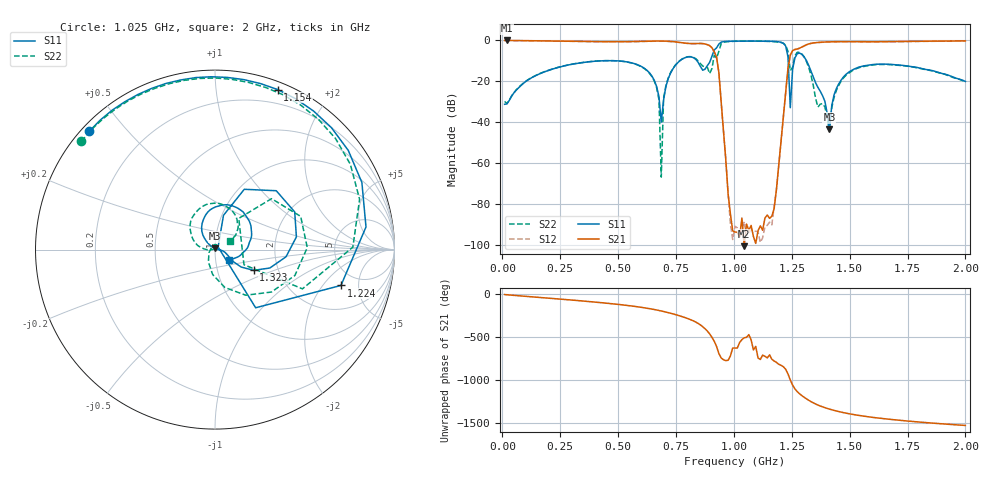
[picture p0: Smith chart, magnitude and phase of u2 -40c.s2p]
!Agilent Technologies,E8363B,SG43030131,A.07.50.48
!Agilent E8363B: A.07.50.48
!Date: Tuesday, December 02, 2025 02:29:57
!Correction: S11(Full 2 Port(1,2))
!S21(Full 2 Port(1,2))
!S12(Full 2 Port(1,2))
!S22(Full 2 Port(1,2))
!S2P File: Measurements: S11, S21, S12, S22:
# Hz S  dB  R 50
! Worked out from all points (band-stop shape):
!   201 points, 10 MHz to 2 GHz, reference 50 ohm
!   highest |S21| = 0.00 dB at 19.95 MHz (marker M1); lowest = -100.8 dB at 1.045 GHz (marker M2)
!   |S21| within 3 dB of the highest: start of sweep to 900.1 MHz; 1.297 GHz to end of sweep
!   lowest |S11| = -43.5 dB at 1.413 GHz (marker M3), VSWR 1.01, Z = 49.9 + j0.662 ohm
!   |S11| at or under -10 dB: start of sweep to 421.7 MHz; 498.7 MHz to 766.5 MHz (267.8 MHz wide, 42.3 % of centre); 1.314 GHz to end of sweep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
!   |S22| runs from -66.9 to -0.4 dB; largest |S21 - S12| = 0.019
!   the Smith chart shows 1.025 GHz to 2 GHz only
!   S11 on the Smith chart (normalised r, x): 1.025 GHz: 0.02, +0.40; 1.154 GHz: 0.07, +1.46; 1.224 GHz: 3.63, -3.10; 1.323 GHz: 1.49, -0.37; 2 GHz: 1.16, -0.14
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1e7  -31.26 -83.7  -0.01 -0.6  -0.08 -1.6  -29.86 -81.1
1.995e7  -31.10 -84.9  0.00 -3.4  -0.08 -4.1  -30.90 -87.6
3.483e8  -10.81 -166.1  -0.47 -76.1  -0.55 -76.1  -10.76 -163.3
6.7665e8  -27.61 91.5  -0.28 173.3  -0.35 173.3  -28.97 86.9
6.866e8  -39.99 135.0  -0.28 167.5  -0.35 167.5  -66.92 -45.5
6.9655e8  -29.17 -128.6  -0.30 161.4  -0.37 161.4  -28.30 -104.4
7.264e8  -16.06 -137.6  -0.46 141.4  -0.53 141.3  -15.84 -123.8
8.5575e8  -12.76 57.1  -1.45 3.8  -1.53 3.7  -11.34 142.2
9.1545e8  -4.66 -116.7  -5.52 172.8  -5.60 172.7  -7.30 -102.7
9.7515e8  -0.43 168.7  -75.05 -48.8  -74.72 -52.8  -0.54 175.7
1.005e9  -0.36 148.2  -93.82 94.1  -91.03 38.0  -0.41 153.0
1.0249e9  -0.34 136.8  -96.21 158.4  -96.09 -58.6  -0.37 141.0
1.0448e9  -0.31 126.3  -100.76 -145.8  -88.77 -97.6  -0.36 130.3
1.15425e9  -0.38 68.6  -87.13 14.7  -88.99 -18.3  -0.48 72.7
1.2239e9  -2.74 -15.9  -24.89 -153.9  -24.94 -154.0  -2.29 1.0
1.2438e9  -32.92 39.8  -7.19 80.6  -7.24 80.5  -14.80 -27.6
1.2637e9  -8.55 64.1  -4.41 -23.0  -4.48 -23.1  -7.46 42.0
1.3234e9  -12.25 -28.3  -1.70 -157.1  -1.78 -157.3  -13.22 -75.3
1.3433e9  -18.08 -33.4  -1.21 172.6  -1.28 172.6  -22.18 -118.3
1.41295e9  -43.45 99.4  -0.67 100.1  -0.74 100.0  -44.36 155.8
1.67165e9  -11.63 53.6  -0.58 -18.7  -0.64 -18.9  -11.81 83.6
2e9  -20.08 -37.0  -0.22 -90.9  -0.28 -91.0  -20.36 29.6
